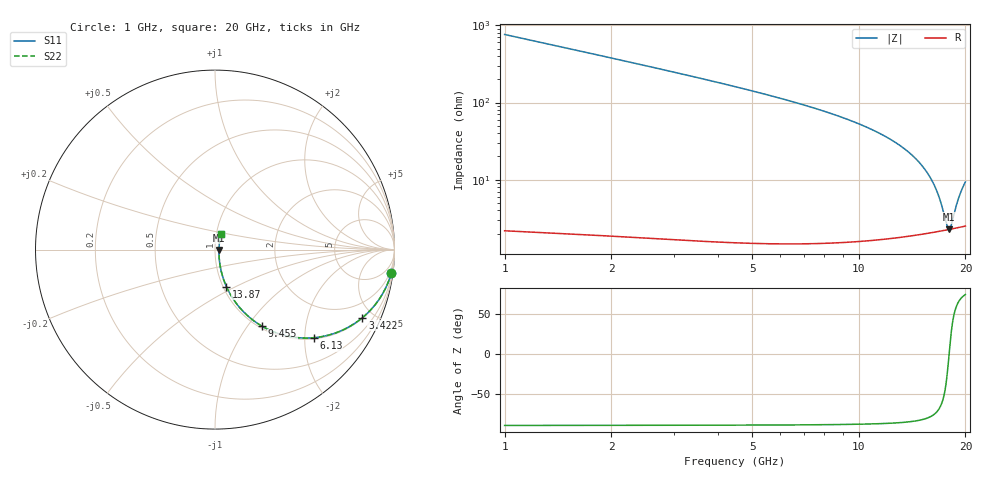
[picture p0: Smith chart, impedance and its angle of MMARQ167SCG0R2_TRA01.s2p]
! MMARQ167SCG0R2_TRA01  S-PARAMETER MODEL  ( General Type )
! Model Generated by TAIYO YUDEN Corporation (http://www.ty-top.com)
! Version 1.0
! TAIYO YUDEN Control No. 180601
! Copyright(c) 2018 TAIYO YUDEN CO.,LTD. All Rights Reserved.
! Product Description (link to TY-COMPAS)
! https://ds.yuden.co.jp/TYCOMPAS/or/detail?pn=MMARQ167SCG0R2ATRA01&u=M
! Products Name : Multilayer Ceramic Capacitors
! Characteristics :
!  Capacitance : 0.2 pF , Rated Voltage : 250V , TCC : CG / C0G
!  Case Size : 1.6 x 0.8 / 0.063 x 0.031 [mm/inch] , Thickness : 0.7 / 0.028 [mm/inch]
!  (Conditions: Temperature = 25 degC , DC Bias Current/Voltage = 0A / 0V)
! External Node Assignments :
!  1  o---| |---o  2
! GND o---------o GND
! Frequency Range : 1000MHz  -  20000MHz  [ 401 STEP ]
# MHz S RI R 50
! Freq[MHz].  S11 Real  S11 Imag  S21 Real  S21 Imag  S12 Real  S12 Imag  S22 Real  S22 Imag
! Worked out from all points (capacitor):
!   401 points, 1 GHz to 20 GHz, reference 50 ohm
!   read as one part in series: C = 208 fF near 1.095 GHz
!   lowest |Z| = 2.26 ohm at 17.96 GHz (marker M1)
!   series resonance near 17.99 GHz, so ESL is about 380 pH
!   S11 on the Smith chart (normalised r, x): 1 GHz: 1, -15; 3.422 GHz: 1.03, -4.31; 6.13 GHz: 1.03, -2.21; 9.455 GHz: 1.03, -1.17; 13.87 GHz: 1.04, -0.45; 20 GHz: 1.05, +0.18
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1000  0.9827 -0.1289  0.0173 0.1289  0.0173 0.1289  0.9827 -0.1289
1522.5  0.9607 -0.1924  0.0393 0.1924  0.0393 0.1924  0.9607 -0.1924
2045  0.9306 -0.2516  0.0694 0.2516  0.0694 0.2516  0.9306 -0.2516
3422.5  0.8212 -0.3795  0.1788 0.3795  0.1788 0.3795  0.8212 -0.3795
4182.5  0.7482 -0.4296  0.2518 0.4296  0.2518 0.4296  0.7482 -0.4296
6130  0.5491 -0.491  0.4509 0.491  0.4509 0.491  0.5491 -0.491
7365  0.4298 -0.4866  0.5702 0.4866  0.5702 0.4866  0.4298 -0.4866
9455  0.2615 -0.4264  0.7385 0.4264  0.7385 0.4264  0.2615 -0.4264
10500  0.1959 -0.3806  0.8041 0.3806  0.8041 0.3806  0.1959 -0.3806
12210  0.1147 -0.2943  0.8853 0.2943  0.8853 0.2943  0.1147 -0.2943
13682.5  0.0679 -0.2158  0.9321 0.2158  0.9321 0.2158  0.0679 -0.2158
13872.5  0.0633 -0.2056  0.9367 0.2056  0.9367 0.2056  0.0633 -0.2056
14822.5  0.0442 -0.1554  0.9558 0.1554  0.9558 0.1554  0.0442 -0.1554
15630  0.0331 -0.1137  0.9669 0.1137  0.9669 0.1137  0.0331 -0.1137
16295  0.027 -0.0803  0.973 0.0803  0.973 0.0803  0.027 -0.0803
16865  0.0237 -0.0525  0.9763 0.0525  0.9763 0.0525  0.0237 -0.0525
17720  0.0219 -0.0123  0.9781 0.0123  0.9781 0.0123  0.0219 -0.0123
17957.5  0.0221 -0.00149  0.9779 0.00149  0.9779 0.00149  0.0221 -0.00149
18195  0.0224 0.00918  0.9776 -0.00918  0.9776 -0.00918  0.0224 0.00918
18812.5  0.0243 0.0362  0.9757 -0.0362  0.9757 -0.0362  0.0243 0.0362
19192.5  0.0262 0.0522  0.9738 -0.0522  0.9738 -0.0522  0.0262 0.0522
20000  0.0318 0.085  0.9682 -0.085  0.9682 -0.085  0.0318 0.085
